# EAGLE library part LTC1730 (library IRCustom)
Linear Tech LTC1730 Lipoly charger By microbuilder.eu
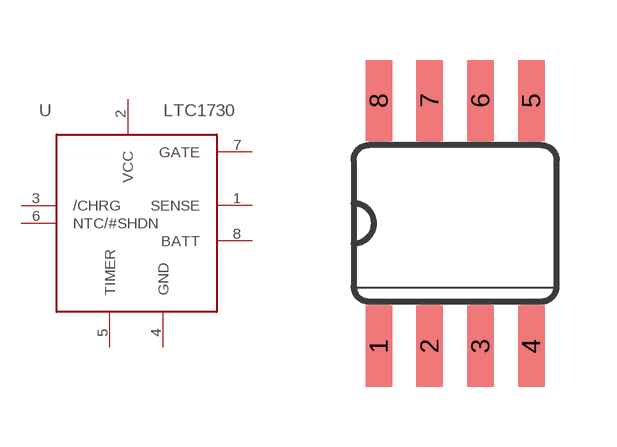
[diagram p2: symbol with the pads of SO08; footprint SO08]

Designator prefix -

## LTC1730  [SO08]
1  SENSE
2  VCC  sup
3  /CHRG
4  GND  sup
5  TIMER  pas
6  NTC/#SHDN  in
7  GATE  out
8  BATT  out

## Footprint SO08 (pad centres in mm)
smd 0.66 x 2.032: 1 -1.905,-3.073; 2 -0.635,-3.073; 3 0.635,-3.073; 4 1.905,-3.073; 5 1.905,3.073; 6 0.635,3.073; 7 -0.635,3.073; 8 -1.905,3.073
